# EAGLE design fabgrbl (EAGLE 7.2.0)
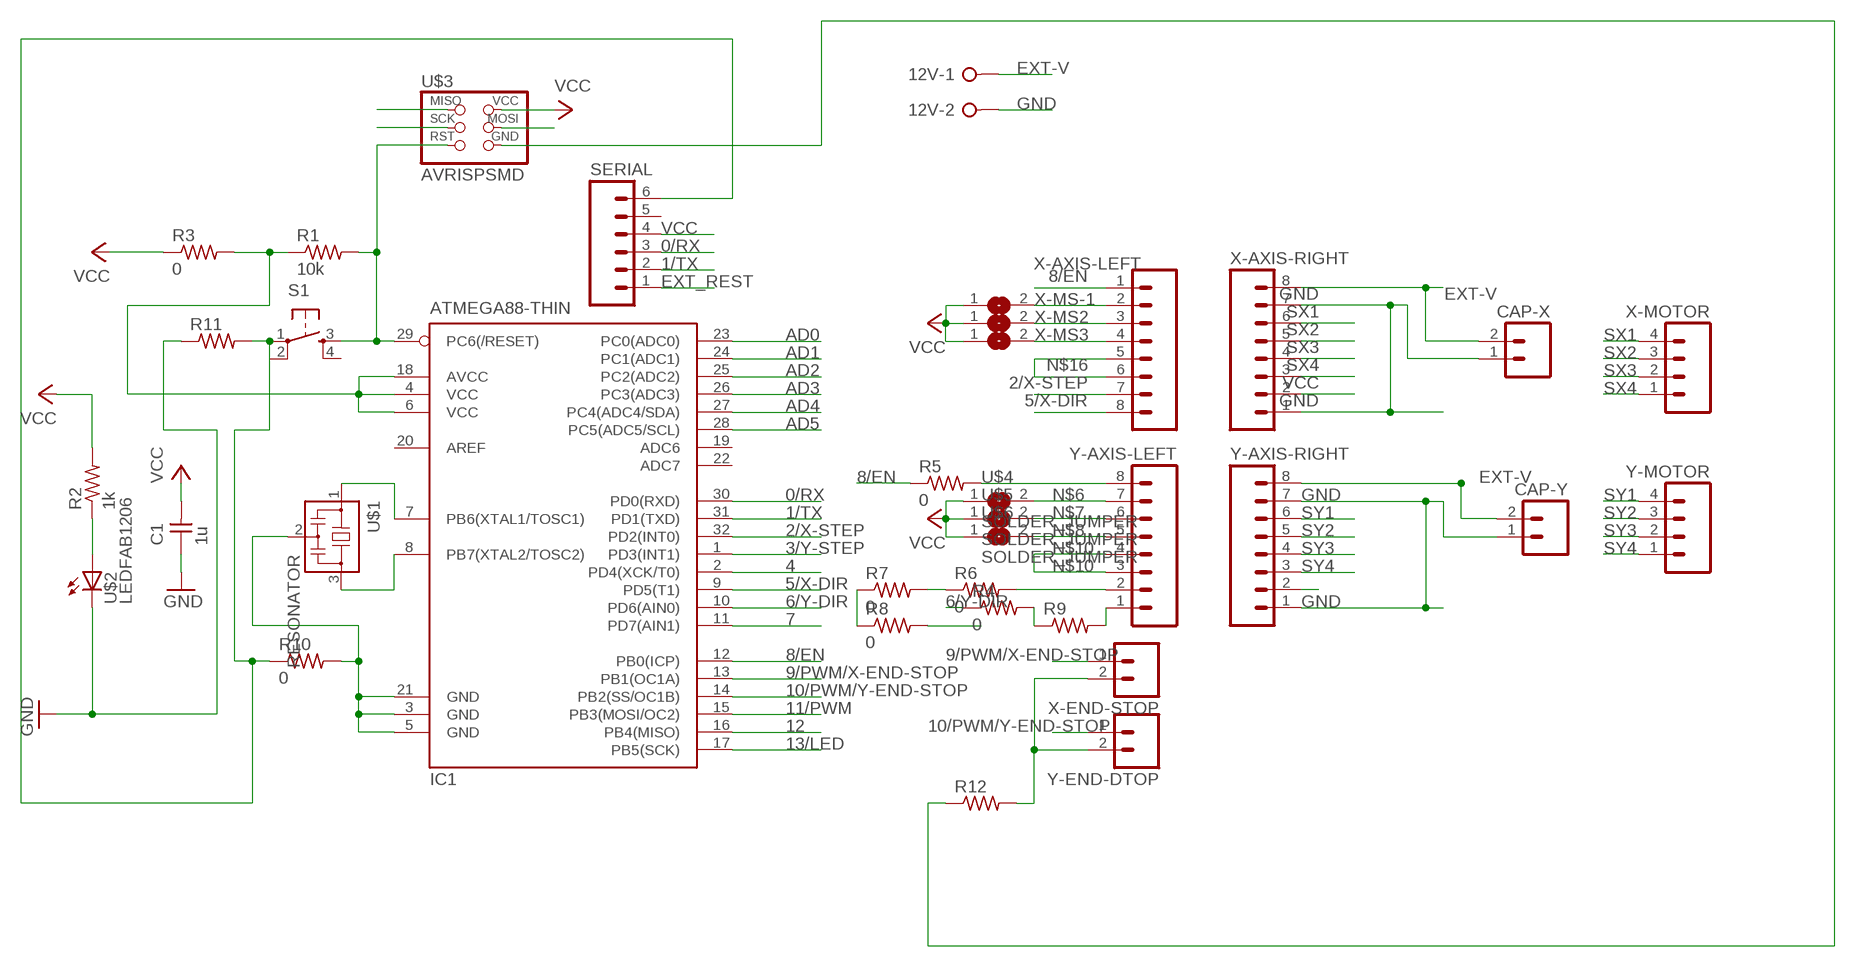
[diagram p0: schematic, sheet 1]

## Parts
12V  W237-02P  [W237-132]
C1  1u  CAP-UNPOLARIZEDFAB  [C1206FAB]
CAP-X  M02LOCK_LONGPADS  [1X02_LOCK_LONGPADS]
CAP-Y  M02LOCK_LONGPADS  [1X02_LOCK_LONGPADS]
IC1  ATMEGA88-THIN  [TQFP32-08THIN]
R1  10k  RES-US1206FAB  [R1206FAB]
R2  1k  RES-US1206FAB  [R1206FAB]
R3  0  RES-US1206FAB  [R1206FAB]
R4  0  RES-US1206FAB  [R1206FAB]
R5  0  RES-US1206FAB  [R1206FAB]
R6  0  RES-US1206FAB  [R1206FAB]
R7  0  RES-US1206FAB  [R1206FAB]
R8  0  RES-US1206FAB  [R1206FAB]
R9  RES-US1206FAB  [R1206FAB]
R10  0  RES-US1206FAB  [R1206FAB]
R11  RES-US1206FAB  [R1206FAB]
R12  RES-US1206FAB  [R1206FAB]
S1  6MM_SWITCH6MM_SWITCH  [6MM_SWITCH]
SERIAL  M06LONGPADS  [1X06_LONGPADS]
U$1  RESONATOR  [EFOBM]
U$2  LEDFAB1206  [LED1206FAB]
U$3  AVRISPSMD  [2X03SMD]
U$4  SOLDER_JUMPER  [SJFAB]
U$5  SOLDER_JUMPER  [SJFAB]
U$6  SOLDER_JUMPER  [SJFAB]
X-AXIS-LEFT  M08LONGPADS  [1X08_LONGPADS]
X-AXIS-RIGHT  M08LONGPADS  [1X08_LONGPADS]
X-END-STOP  M02LOCK_LONGPADS  [1X02_LOCK_LONGPADS]
X-MOTOR  M04LONGPADS  [1X04_LONGPADS]
X-MS2  SOLDER_JUMPER  [SJFAB]
X-MS3  SOLDER_JUMPER  [SJFAB]
X-MS-1  SOLDER_JUMPER  [SJFAB]
Y-AXIS-LEFT  M08LONGPADS  [1X08_LONGPADS]
Y-AXIS-RIGHT  M08LONGPADS  [1X08_LONGPADS]
Y-END-DTOP  M02LOCK_LONGPADS  [1X02_LOCK_LONGPADS]
Y-MOTOR  M04LONGPADS  [1X04_LONGPADS]

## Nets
0/RX: IC1.30(PD0(RXD)) SERIAL.3
1/TX: IC1.31(PD1(TXD)) SERIAL.2
2/X-STEP: IC1.32(PD2(INT0)) X-AXIS-LEFT.7
3/Y-STEP: IC1.1(PD3(INT1)) R8.2
4: IC1.2(PD4(XCK/T0))
5/X-DIR: IC1.9(PD5(T1)) X-AXIS-LEFT.8
6/Y-DIR: IC1.10(PD6(AIN0)) R4.1
7: IC1.11(PD7(AIN1))
8/EN: IC1.12(PB0(ICP)) R5.1 X-AXIS-LEFT.1
9/PWM/X-END-STOP: IC1.13(PB1(OC1A)) X-END-STOP.1
10/PWM/Y-END-STOP: IC1.14(PB2(SS/OC1B)) Y-END-DTOP.1
11/PWM: IC1.15(PB3(MOSI/OC2)) U$3.4(MOSI)
12: IC1.16(PB4(MISO)) U$3.1(MISO)
13/LED: IC1.17(PB5(SCK)) U$3.3(SCK)
AD0: IC1.23(PC0(ADC0))
AD1: IC1.24(PC1(ADC1))
AD2: IC1.25(PC2(ADC2))
AD3: IC1.26(PC3(ADC3))
AD4: IC1.27(PC4(ADC4/SDA))
AD5: IC1.28(PC5(ADC5/SCL))
EXT-V: 12V.1 CAP-X.2 CAP-Y.2 X-AXIS-RIGHT.8 Y-AXIS-RIGHT.8
EXT_REST: SERIAL.1
GND: 12V.2 C1.1 CAP-X.1 CAP-Y.1 R11.1 U$2.2(C) X-AXIS-RIGHT.1 X-AXIS-RIGHT.7 Y-AXIS-RIGHT.1 Y-AXIS-RIGHT.7
N$1: IC1.7(PB6(XTAL1/TOSC1)) U$1.1
N$2: IC1.8(PB7(XTAL2/TOSC2)) U$1.3
N$3: R10.1 R11.2 S1.1(P)
N$4: R2.1 U$2.1(A)
N$5: R5.2 Y-AXIS-LEFT.8
N$6: U$4.2 Y-AXIS-LEFT.7
N$7: U$5.2 Y-AXIS-LEFT.6
N$8: U$6.2 Y-AXIS-LEFT.5
N$9: R9.2 Y-AXIS-LEFT.1
N$10: Y-AXIS-LEFT.3 Y-AXIS-LEFT.4
N$11: R6.2 Y-AXIS-LEFT.2
N$12: R6.1 R7.2
N$13: IC1.29(PC6(/RESET)) R1.2 S1.3(S) U$3.5(RST)
N$14: R7.1 R8.1
N$15: R4.2 R9.1
N$16: X-AXIS-LEFT.5 X-AXIS-LEFT.6
N$17: X-AXIS-LEFT.4 X-MS3.2
N$18: X-AXIS-LEFT.3 X-MS2.2
N$19: X-AXIS-LEFT.2 X-MS-1.2
N$20: IC1.4(VCC) IC1.6(VCC) IC1.18(AVCC) R1.1 R3.2
N$21: SERIAL.6
N$22: IC1.3(GND) IC1.5(GND) IC1.21(GND) R10.2 U$1.2
N$23: R12.2 X-END-STOP.2 Y-END-DTOP.2
N$24: R12.1 U$3.6(GND)
SX1: X-AXIS-RIGHT.6 X-MOTOR.4
SX2: X-AXIS-RIGHT.5 X-MOTOR.3
SX3: X-AXIS-RIGHT.4 X-MOTOR.2
SX4: X-AXIS-RIGHT.3 X-MOTOR.1
SY1: Y-AXIS-RIGHT.6 Y-MOTOR.4
SY2: Y-AXIS-RIGHT.5 Y-MOTOR.3
SY3: Y-AXIS-RIGHT.4 Y-MOTOR.2
SY4: Y-AXIS-RIGHT.3 Y-MOTOR.1
VCC: C1.2 R2.2 R3.1 SERIAL.4 U$3.2(VCC) U$4.1 U$5.1 U$6.1 X-AXIS-RIGHT.2 X-MS2.1 X-MS3.1 X-MS-1.1 Y-AXIS-RIGHT.2
Unconnected: IC1.19(ADC6) IC1.20(AREF) IC1.22(ADC7) S1.2(P1) S1.4(S1) SERIAL.5

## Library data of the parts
12V = con-wago-508:W237-02P: WAGO SREW CLAMP; OC_FARNELL: unknown; OC_NEWARK: unknown
C1 = fab:CAP-UNPOLARIZED
CAP-X CAP-Y X-END-STOP Y-END-DTOP = SparkFun-Connectors:M02: Standard 2-pin 0.1" header. Use with
IC1 = fab:ATMEGA88-THIN
R1-R12 = fab:RES-US: Resistor (US Symbol)
S1 = fab:6MM_SWITCH: OMRON SWITCH
SERIAL = SparkFun-Connectors:M06: Header 6 Standard 6-pin 0.1" header. Use with straight break away headers (SKU : PRT-00116), right angle break away headers (PRT-00553), swiss pins (PRT-00743), machine pins (PRT-00117), and female headers (PRT-00115). Molex polarized connector foot print use with SKU : PRT-08094 with associated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
U$1 = fab:RESONATOR
U$2 = fab:LED: LED
U$3 = fab:AVRISP
U$4-U$6 X-MS2 X-MS3 X-MS-1 = fab:SOLDER_JUMPER
X-AXIS-LEFT X-AXIS-RIGHT Y-AXIS-LEFT Y-AXIS-RIGHT = SparkFun-Connectors:M08: Header 8 Standard 8-pin 0.1" header. Use with straight break away headers (SKU : PRT-00116), right angle break away headers (PRT-00553), swiss pins (PRT-00743), machine pins (PRT-00117), and female headers (PRT-00115).
X-MOTOR Y-MOTOR = SparkFun-Connectors:M04: Header 4 Standard 4-pin 0.1" header. Use with straight break away headers (SKU : PRT-00116), right angle break away headers (PRT-00553), swiss pins (PRT-00743), machine pins (PRT-00117), and female headers (PRT-00115). Molex polarized connector foot print use with SKU : PRT-08231 with associated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

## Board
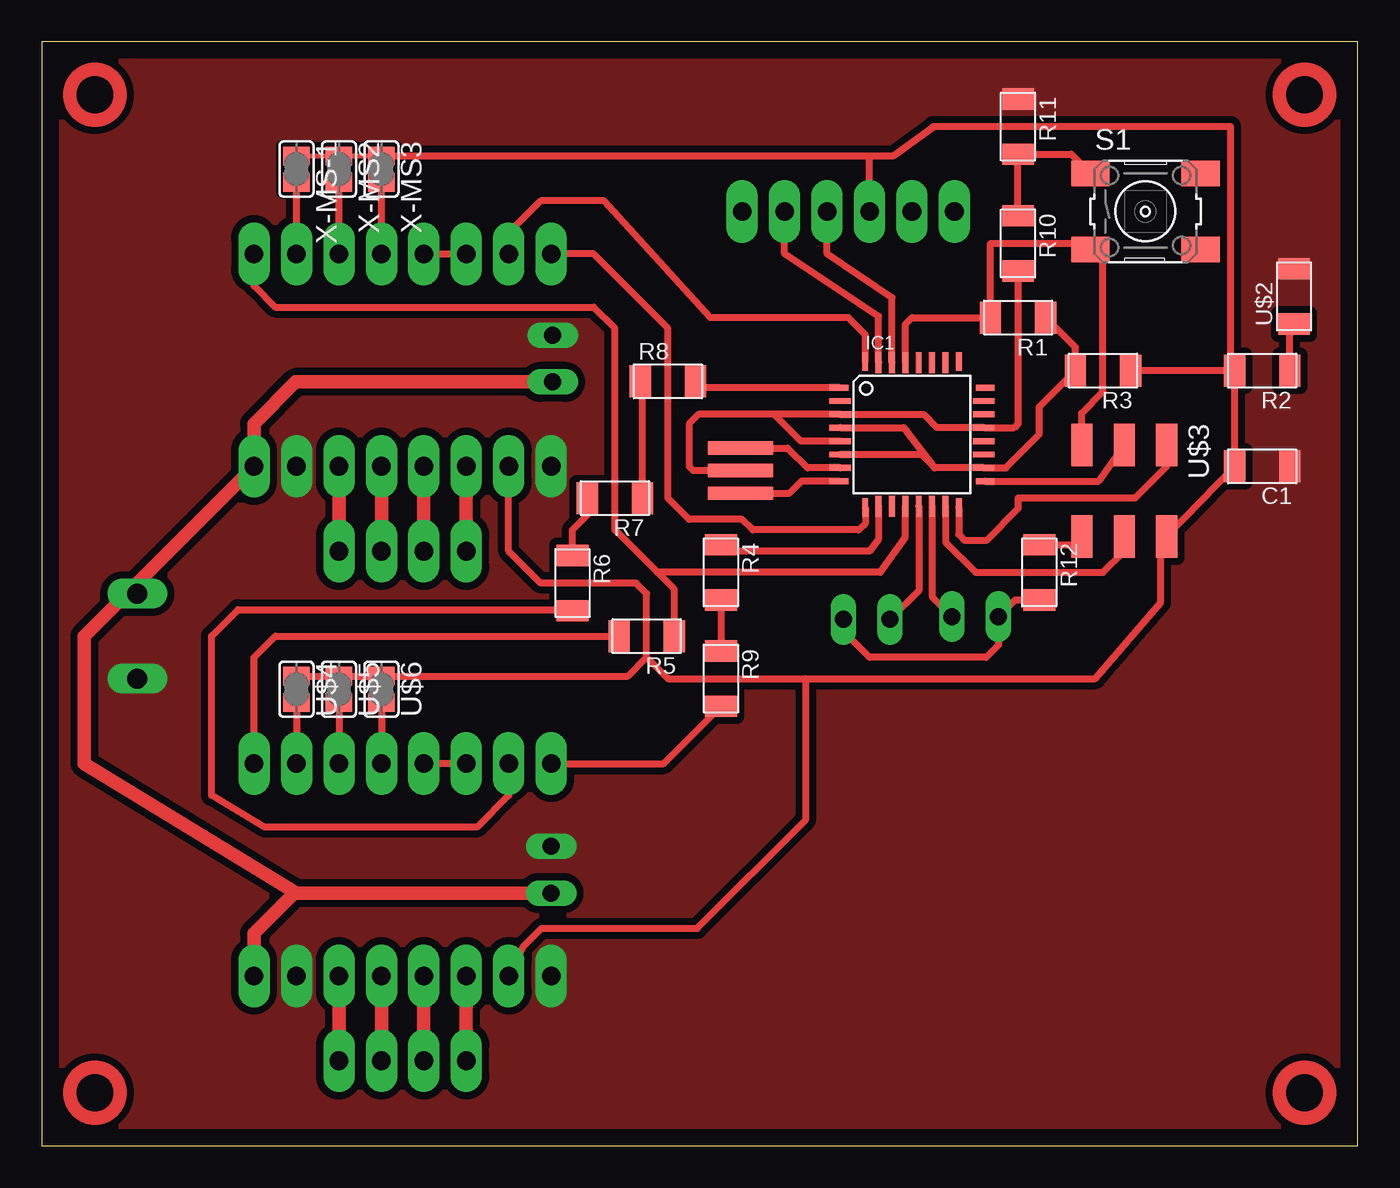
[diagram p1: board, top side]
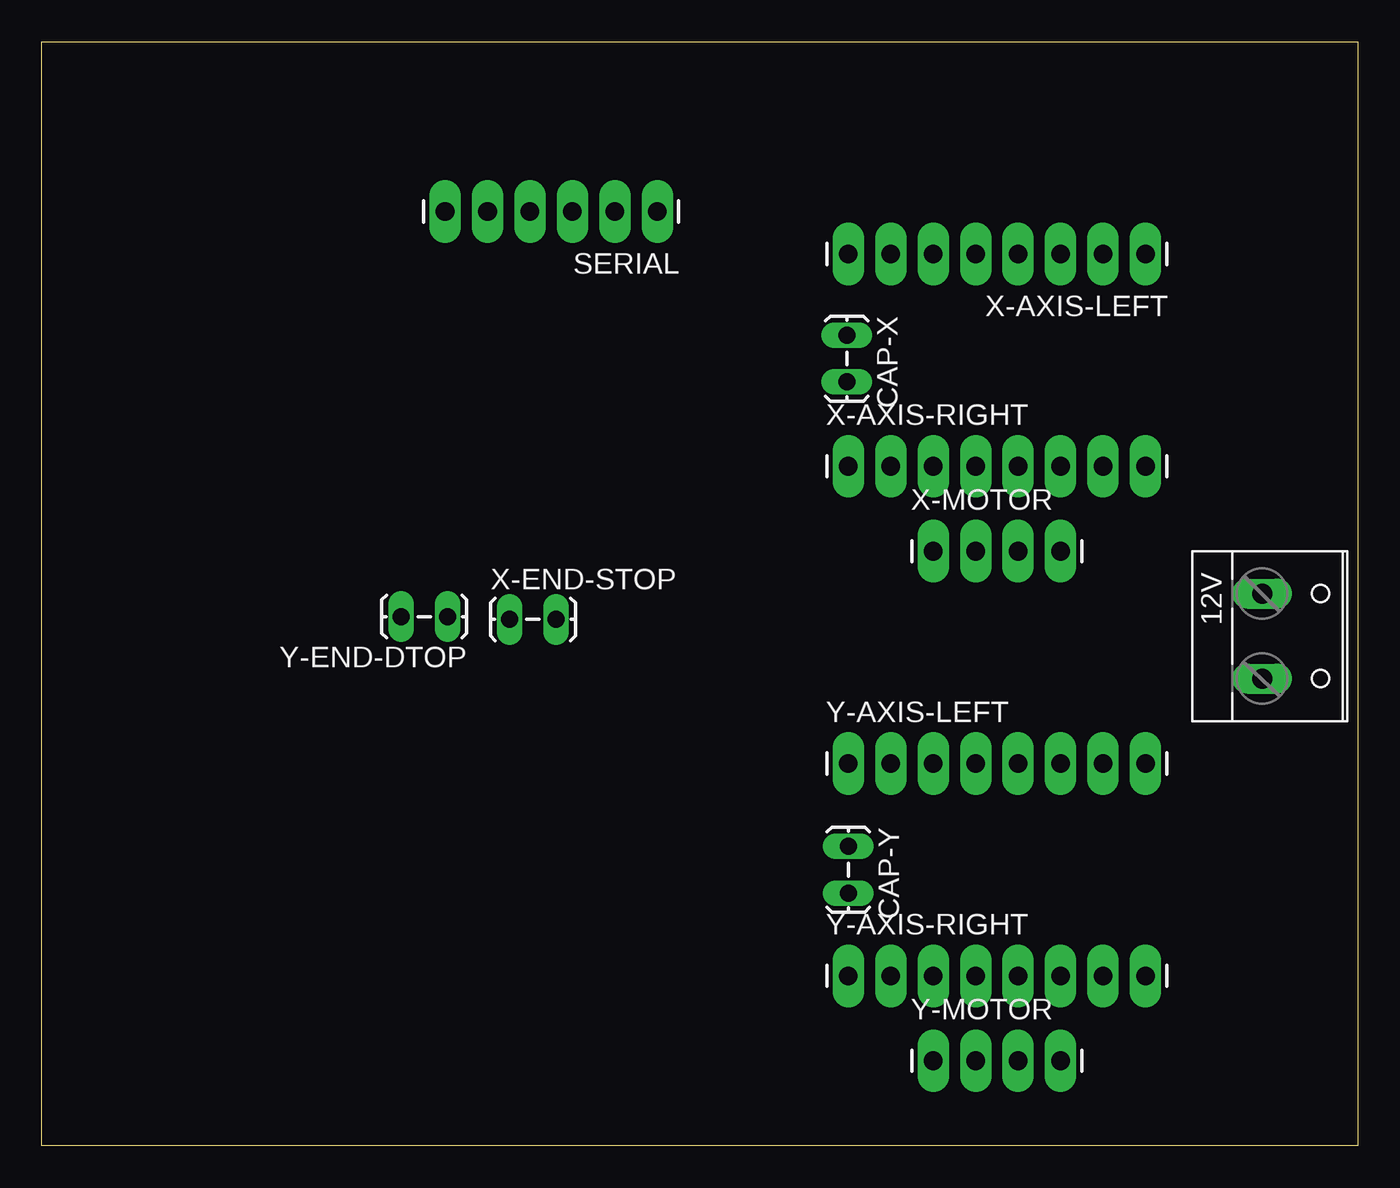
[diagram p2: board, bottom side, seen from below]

Size 78.74 x 66.03 mm. Coordinates in mm from the lower left corner, seen from the top.
Outline: 0,0 78.74,0 78.74,66.03 0,66.03 0,0
Copper layers (1*16): Top 0.035mm / dielectric 1.5mm / Bottom 0.035mm
Design rules "default *": minimum track width 10mil, minimum drill 24mil, track to track 17mil, track to pad 17mil, pad to pad 17mil, via to via 17mil, smd to smd 17mil, copper to edge 40mil, drill to drill 8mil, minimum pad ring 10mil, minimum via ring 8mil, stop-mask expansion 4mil, vias tented up to drill 0mil, thermal gap 10mil

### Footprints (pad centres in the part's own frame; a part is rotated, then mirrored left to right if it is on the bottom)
W237-132 = drill 1.194 long: 1 -2.54,-0.635; 2 2.54,-0.635
C1206FAB = smd 1.27 x 1.905: 1 -1.651,0; 2 1.651,0
1X02_LOCK_LONGPADS = drill 1.016 long: 1 -0.127,0; 2 2.667,0
TQFP32-08THIN = smd 1.118 x 0.356: 1 -4.369,2.8; 8 -4.369,-2.8; 17 4.369,-2.8; 24 4.369,2.8 | smd 1.27 x 0.356: 2 -4.293,2; 3 -4.293,1.2; 4 -4.293,0.4; 5 -4.293,-0.4; 6 -4.293,-1.2; 7 -4.293,-2; 18 4.293,-2; 19 4.293,-1.2; 20 4.293,-0.4; 21 4.293,0.4; 22 4.293,1.2; 23 4.293,2 | smd 0.356 x 1.118: 9 -2.8,-4.369; 16 2.8,-4.369; 25 2.8,4.369; 32 -2.8,4.369 | smd 0.356 x 1.27: 10 -2,-4.293; 14 1.2,-4.293; 15 2,-4.293; 26 2,4.293; 27 1.2,4.293; 31 -2,4.293 | smd 0.35 x 1.27: 11 -1.2,-4.293; 12 -0.4,-4.293; 13 0.4,-4.293; 28 0.4,4.293; 29 -0.4,4.293; 30 -1.2,4.293
R1206FAB = smd 1.27 x 1.905: 1 -1.651,0; 2 1.651,0
6MM_SWITCH = smd 2.286 x 1.524: 1 -3.302,2.286; 2 3.302,2.286; 3 -3.302,-2.286; 4 3.302,-2.286
1X06_LONGPADS = drill 1.118 pad 1.88 long: 1 0,0; 2 2.54,0; 3 5.08,0; 4 7.62,0; 5 10.16,0; 6 12.7,0
EFOBM = smd 0.8 x 3.9: 1 -1.35,0; 2 0,0; 3 1.35,0
LED1206FAB = smd 1.27 x 1.905: 1 -1.651,0; 2 1.651,0
2X03SMD = smd 2.54 x 1.27: 1 -2.54,2.54; 2 2.92,2.54; 3 -2.54,0; 4 2.92,0; 5 -2.54,-2.54; 6 2.92,-2.54
SJFAB = smd 1.118 x 1.6: 1 -0.787,0; 2 0.787,0
1X08_LONGPADS = drill 1.118 pad 1.88 long: 1 0,0; 2 2.54,0; 3 5.08,0; 4 7.62,0; 5 10.16,0; 6 12.7,0; 7 15.24,0; 8 17.78,0
1X04_LONGPADS = drill 1.118 pad 1.88 long: 1 0,0; 2 2.54,0; 3 5.08,0; 4 7.62,0

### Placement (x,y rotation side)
12V  5.08,30.48 270 bottom
C1  73.03,40.64 180 top
CAP-X  30.57,48.35 270 bottom
CAP-Y  30.48,17.78 270 bottom
IC1  52.07,42.55 0 top
R1  58.42,49.53 180 top
R2  73.03,46.35 180 top
R3  63.5,46.35 180 top
R4  40.64,34.29 270 top
R5  36.2,30.48 180 top
R6  31.75,33.66 270 top
R7  34.29,38.73 180 top
R8  37.47,45.72 0 top
R9  40.64,27.94 270 top
R10  58.42,53.98 270 top
R11  58.42,60.96 270 top
R12  59.69,34.29 270 top
S1  66.04,55.88 0 top
SERIAL  41.91,55.88 180 bottom
U$1  41.8,40.38 270 top
U$2  74.93,50.8 90 top
U$3  64.77,39.37 270 top
U$4  15.24,27.3 270 top
U$5  17.78,27.3 270 top
U$6  20.32,27.3 270 top
X-AXIS-LEFT  12.7,53.34 180 bottom
X-AXIS-RIGHT  30.48,40.64 0 bottom
X-END-STOP  50.62,31.49 0 bottom
X-MOTOR  25.4,35.56 0 bottom
X-MS2  17.78,58.42 270 top
X-MS3  20.32,58.42 270 top
X-MS-1  15.24,58.42 270 top
Y-AXIS-LEFT  30.48,22.86 0 bottom
Y-AXIS-RIGHT  30.48,10.16 0 bottom
Y-END-DTOP  54.58,31.65 180 bottom
Y-MOTOR  25.4,5.08 0 bottom

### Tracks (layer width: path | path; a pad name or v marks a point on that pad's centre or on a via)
0/RX
  Top 0.406: IC1.30 50.87,50.73 46.99,53.34 SERIAL.3
1/TX
  Top 0.406: IC1.31 50.07,49.62 44.45,53.34 SERIAL.2
2/X-STEP
  Top 0.406: IC1.32 49.27,48.52 48.26,49.53 40.01,49.53 33.66,56.52 29.84,56.52 27.94,54.61 X-AXIS-LEFT.7
3/Y-STEP
  Top 0.406: IC1.1 41.53,45.34 39.49,45.34 R8.2
5/X-DIR
  Top 0.406: IC1.9 49.27,37.2 48.9,36.83 42.55,36.83 41.91,37.47 38.73,37.47 37.47,38.73 37.47,48.9 33.02,53.34 X-AXIS-LEFT.8
6/Y-DIR
  Top 0.406: IC1.10 50.07,36.29 49.53,35.56 41.02,35.56 R4.1
8/EN
  Top 0.406: R5.1 37.85,33.27 36.83,34.29 | 36.83,34.29 34.29,36.83 34.29,48.9 33.02,50.16 13.97,50.16 12.7,51.44 X-AXIS-LEFT.1 | 36.83,34.29 50.16,34.29 51.67,36.43 IC1.12
9/PWM/X-END-STOP
  Top 0.406: IC1.13 52.47,33.21 X-END-STOP.1
10/PWM/Y-END-STOP
  Top 0.406: IC1.14 53.27,32.84 Y-END-DTOP.1
11/PWM
  Top 0.305: 64.77,35.56 U$3.4
  Top 0.406: 64.35,36.4 U$3.4 | IC1.15 54.07,36.1 55.88,34.29 63.5,34.29 64.77,35.56
12
  Top 0.406: IC1.16 54.87,36.57 55.24,36.2 56.52,36.2 58.42,38.1 58.42,38.73 65.41,38.73 67.31,40.64 U$3.1
13/LED
  Top 0.406: IC1.17 63.24,39.74 U$3.3
EXT-V
  Top 0.813: CAP-Y.2 15.24,15.11 | 15.24,15.11 15.11,15.11 12.7,12.7 Y-AXIS-RIGHT.8 | 12V.1 5.08,33.02 | 5.08,33.02 2.54,30.48 2.54,22.86 15.24,15.11 | CAP-X.2 15.2,45.68 12.7,43.18 X-AXIS-RIGHT.8 5.08,33.02
GND
  pour Top (isolate 0.406, no thermals): 0.01,0 78.74,0 78.74,66.04 0,66.04
N$1
  Top 0.406: U$1.1 44.63,41.73 45.81,40.55 IC1.7
N$2
  Top 0.406: IC1.8 45.46,39.74 44.74,39.03 U$1.3
N$3
  Top 0.406: R10.1 R11.2 61.59,59.31 S1.1
N$4
  Top 0.305: U$2.1 75.44,49.29
  Top 0.406: R2.1 74.68,48.53 75.44,49.29
N$5
  Top 0.406: Y-AXIS-LEFT.8 12.7,29.21 13.97,30.48 R5.2
N$6
  Top 0.406: U$4.2 Y-AXIS-LEFT.7
N$7
  Top 0.406: U$5.2 Y-AXIS-LEFT.6
N$8
  Top 0.406: U$6.2 Y-AXIS-LEFT.5
N$9
  Top 0.406: Y-AXIS-LEFT.1 37.21,22.86 R9.2
N$10
  Top 0.406: Y-AXIS-LEFT.3 Y-AXIS-LEFT.4
N$11
  Top 0.406: Y-AXIS-LEFT.2 27.94,20.95 26.04,19.05 13.34,19.05 10.16,20.95 10.16,30.48 11.75,32.07 31.75,32.07 R6.2
N$12
  Top 0.406: R6.1 31.75,36.83 33.02,38.1 33.02,38.35 R7.2
N$13
  Top 0.406: IC1.29 51.67,49.13 52.07,49.53 R1.2 56.77,53.98 62.74,53.98 S1.3 63.5,53.59 63.5,45.09 62.23,43.81 U$3.5
N$14
  Top 0.406: R7.1 35.94,45.72 R8.1
N$15
  Top 0.406: R4.2 R9.1
N$16
  Top 0.406: X-AXIS-LEFT.5 X-AXIS-LEFT.6
N$17
  Top 0.406: X-AXIS-LEFT.4 X-MS3.2
N$18
  Top 0.406: X-AXIS-LEFT.3 X-MS2.2
N$19
  Top 0.406: X-AXIS-LEFT.2 X-MS-1.2
N$20
  Top 0.254: 53.44,40.55 53.34,40.64
  Top 0.406: IC1.4 51.57,42.95 51.74,42.78 53.44,40.55 IC1.18 57.69,40.55 59.69,42.55 59.69,44.2 R3.2 61.85,47.75 R1.1 | IC1.6 52.63,41.34 53.34,40.64
N$22
  Top 0.406: R10.2 58.42,43.18 58.19,42.95 IC1.21 53.58,42.95 52.77,43.74 IC1.3 43.81,43.74 | 43.81,43.74 39.3,43.74 38.73,43.18 38.73,40.64 38.99,40.38 U$1.2 | IC1.5 45.41,42.15 43.81,43.74
N$23
  Top 0.406: R12.2 58.23,32.64 Y-END-DTOP.2 57.25,29.94 56.52,29.21 49.53,29.21 48.26,30.48 48.26,31.18 X-END-STOP.2
N$24
  Top 0.406: R12.1 61.72,35.94 U$3.6
SX1
  Top 0.813: X-AXIS-RIGHT.6 X-MOTOR.4
SX2
  Top 0.813: X-AXIS-RIGHT.5 X-MOTOR.3
SX3
  Top 0.813: X-AXIS-RIGHT.4 X-MOTOR.2
SX4
  Top 0.813: X-AXIS-RIGHT.3 X-MOTOR.1
SY1
  Top 0.813: Y-MOTOR.4 Y-AXIS-RIGHT.6
SY2
  Top 0.813: Y-MOTOR.3 Y-AXIS-RIGHT.5
SY3
  Top 0.813: Y-MOTOR.2 Y-AXIS-RIGHT.4
SY4
  Top 0.813: Y-MOTOR.1 Y-AXIS-RIGHT.3
VCC
  Top 0.305: 71.12,46.61 R2.2 | X-MS-1.1 X-MS2.1 X-MS3.1 | 66.95,36.09 U$3.2
  Top 0.406: Y-AXIS-RIGHT.2 28.87,11.97 29.9,13 39.22,13 45.72,19.5 45.72,27.94 | U$4.1 U$5.1 U$6.1 35.08,28.09 36.2,29.21 | 36.2,29.21 37.47,27.94 45.72,27.94 | 36.2,29.21 36.2,33.02 35.56,33.66 29.84,33.66 27.94,35.56 X-AXIS-RIGHT.2 | U$3.2 C1.2 R2.2 R3.1 | 71.12,46.61 71.12,60.96 53.34,60.96 50.95,59.21 50.8,59.21 49.53,59.21 | X-MS3.1 49.53,59.21 | 66.95,36.09 66.95,32.5 63.05,27.96 63.05,27.94 45.72,27.94 | SERIAL.4 49.53,59.21
(copper drawn outside any net)
  shapes: Top circle x4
